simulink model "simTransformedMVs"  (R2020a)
settings: Solver=VariableStepAuto  StartTime=0.0  StopTime=tsim  RelTol=1e-3
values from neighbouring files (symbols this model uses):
  p = [V;A(i);B(i)]    [runTransformedMVs.m]    (also in runTransformedMVsIS.m; Main.m = [N, Fc0, rhoc, rhoh,U,A,cpc,cph]; Main_OL.m = [N, Fc0, rhoc, rhoh,U,A,cpc,cph]; runTestCalcBlk.m = [N, Fc0, rhoc, rhoh,U,A,cpc,cph])
  q1max = 10    [runTransformedMVs.m]    (also in runTransformedMVsIS.m)
  q2max = 10    [runTransformedMVs.m]    (also in runTransformedMVsIS.m)
  qmin = 0    [runTransformedMVs.m]    (also in runTransformedMVsIS.m = -inf)
  T0 = 35    [runTransformedMVs.m]    (also in runTransformedMVsIS.m; H2P_Turbine_driven.m = param(9); runTD.m = 318; H2P_Boiler_driven.m = param(9))
  T10 = 20    [runTransformedMVs.m]    (also in runTransformedMVsIS.m)
  T1f = T10-5    (= 15)    [runTransformedMVs.m]    (also in runTransformedMVsIS.m = 25)
  T1fm = T10    (= 20)    [runTransformedMVs.m]    (also in runTransformedMVsIS.m = 25)
  T20 = 50    [runTransformedMVs.m]    (also in runTransformedMVsIS.m)
  T2f = T20    (= 50)    [runTransformedMVs.m]    (also in runTransformedMVsIS.m = 70)
  T2fm = T20    (= 50)    [runTransformedMVs.m]    (also in runTransformedMVsIS.m = 70)
  td1 = 100    [runTransformedMVs.m]    (also in runTransformedMVsIS.m = 200)
  td2 = 150    [runTransformedMVs.m]    (also in runTransformedMVsIS.m = 300)
  tv1 = 50    [runTransformedMVs.m]    (also in runTransformedMVsIS.m = 100)
  tv2 = 50    [runTransformedMVs.m]    (also in runTransformedMVsIS.m = 100)
  v10 = q0    (= 10)    [runTransformedMVs.m]    (also in runTransformedMVsIS.m)
  v1f = q0    (= 10)    [runTransformedMVs.m]    (also in runTransformedMVsIS.m = 15)
  v20 = B(i)^(-1)*(f20-A(i)*T0)    [runTransformedMVs.m]    (also in runTransformedMVsIS.m; runTransfOL.m = v00)
  v2f = v20    [runTransformedMVs.m]    (also in runTransformedMVsIS.m)
undefined symbols (not defined in the file or in its folder): InputTransfD, InvInputTransfD, TempMixDAE

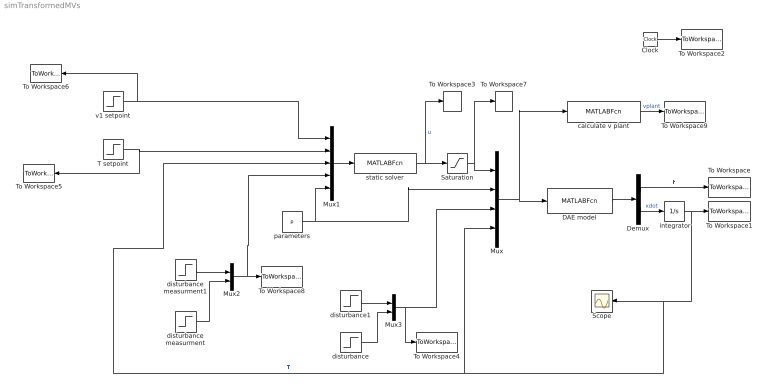
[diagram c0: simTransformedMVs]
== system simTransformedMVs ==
  " integrator" : Integrator  InitialCondition=T0
  Clock : Clock
  DAE model : MATLABFcn  MATLABFcn=TempMixDAE(u(1:2), u(3:5),u(6:7),u(8))  OutputDimensions=2
  Demux : Demux  Outputs=2
  Mux : Mux
  Mux1 : Mux  Inputs=5
  Mux2 : Mux  Inputs=2
  Mux3 : Mux  Inputs=2
  Saturation : Saturate  UpperLimit=[q1max;q2max]  LowerLimit=[qmin;qmin]
  Scope : Scope
  T setpoint : Step  Time=tv2  Before=v20  After=v2f  SampleTime=0
  To Workspace : ToWorkspace  VariableName=q  SampleTime=-1
  To Workspace1 : ToWorkspace  VariableName=T  SampleTime=-1
  To Workspace2 : ToWorkspace  VariableName=time  SampleTime=-1
  To Workspace3 : ToWorkspace  VariableName=u  SampleTime=-1
  To Workspace4 : ToWorkspace  VariableName=d  SampleTime=-1
  To Workspace5 : ToWorkspace  VariableName=v2s  SampleTime=-1
  To Workspace6 : ToWorkspace  VariableName=v1s  SampleTime=-1
  To Workspace7 : ToWorkspace  VariableName=uplant  SampleTime=-1
  To Workspace8 : ToWorkspace  VariableName=dm  SampleTime=-1
  To Workspace9 : ToWorkspace  VariableName=v  SampleTime=-1
  calculate v plant : MATLABFcn  MATLABFcn=InputTransfD(u(1:2),u(3:5),u(6:7),u(8))  OutputDimensions=2
  disturbance : Step  Time=td2  Before=T20  After=T2f  SampleTime=0
  disturbance measurment : Step  Time=td2  Before=T20  After=T2fm  SampleTime=0
  disturbance measurment1 : Step  Time=td1  Before=T10  After=T1fm  SampleTime=0
  disturbance1 : Step  Time=td1  Before=T10  After=T1f  SampleTime=0
  parameters : Constant  Value=p
  static solver : MATLABFcn  MATLABFcn=InvInputTransfD(u(1:2),u(3),u(4:5),u(6:8))  OutputDimensions=2
  v1 setpoint : Step  Time=tv1  Before=v10  After=v1f  SampleTime=0
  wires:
  DAE model/1 -> Demux/1
  Demux/1 -> To Workspace/1  "F"
  " integrator"/1 -> To Workspace1/1, Scope/1, Mux/4, Mux1/3  "T"
  Mux/1 -> calculate v plant/1, DAE model/1
  Clock/1 -> To Workspace2/1
  T setpoint/1 -> Mux1/2, To Workspace5/1
  Mux1/1 -> static solver/1
  v1 setpoint/1 -> Mux1/1, To Workspace6/1
  Demux/2 -> " integrator"/1  "xdot"
  parameters/1 -> Mux/2, Mux1/5
  disturbance/1 -> Mux3/2
  static solver/1 -> Saturation/1, To Workspace3/1  "u"
  Saturation/1 -> To Workspace7/1, Mux/1
  Mux2/1 -> Mux1/4, To Workspace8/1
  calculate v plant/1 -> To Workspace9/1  "vplant"
  disturbance measurment1/1 -> Mux2/1
  disturbance measurment/1 -> Mux2/2
  disturbance1/1 -> Mux3/1
  Mux3/1 -> To Workspace4/1, Mux/3
